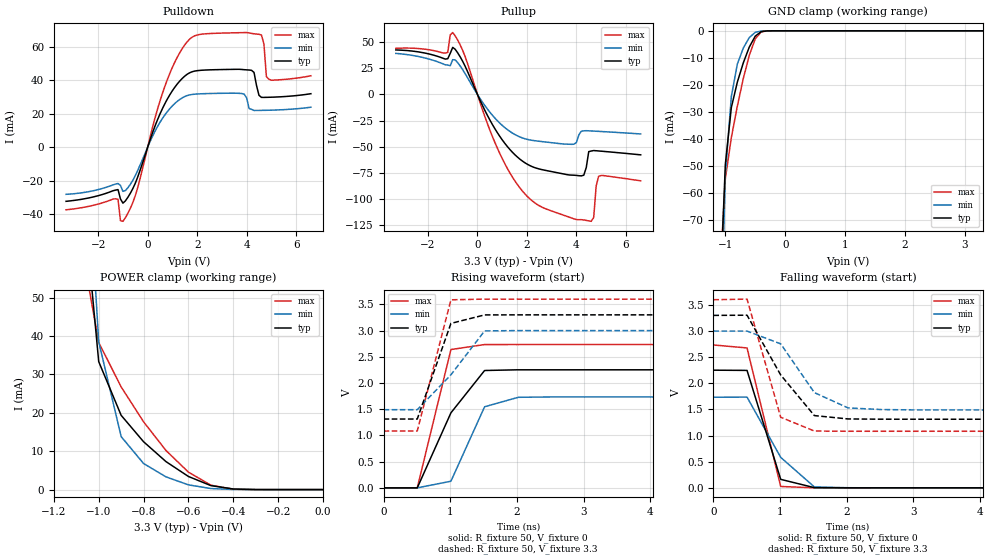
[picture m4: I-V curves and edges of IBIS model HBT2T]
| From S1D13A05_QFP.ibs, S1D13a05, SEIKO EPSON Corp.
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[Model]   HBT2T
Model_type I/O
Enable Active-Low
Polarity Non-Inverting
Vinh=2.0
Vinl=0.8
Vref=0
Vmeas=1.65
Rref=500
Cref=100pf
C_comp   5p   4p   6p
[Temperature Range] 25   85   -40
[Voltage Range]   3.3   3.0   3.6
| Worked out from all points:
|   slope of the pulldown table from 0 to 0.495 V, typ, clamps not added: 25.1 ohm
|   slope of the pullup table from 0 to 0.495 V, typ, clamps not added: 20.5 ohm
|   GND clamp passes 1 mA (typ) near -0.44 V on its own axis
|   POWER clamp passes 1 mA (typ) near -0.50 V on its own axis
|   falling waveform, R_fixture 50, V_fixture 0: 20-80 % time 327ps typ, 563ps min, 313ps max; typ from 2.25 V to 0 V
|   falling waveform, R_fixture 50, V_fixture 3.3: 20-80 % time 620ps typ, 525ps min, 337ps max; typ from 3.3 V to 1.31 V
|   rising waveform, R_fixture 50, V_fixture 0: 20-80 % time 578ps typ, 370ps min, 314ps max; typ from 0 V to 2.25 V
|   rising waveform, R_fixture 50, V_fixture 3.3: 20-80 % time 330ps typ, 603ps min, 305ps max; typ from 1.31 V to 3.3 V
[Pullup]
-3.3V     42.64mA    39.34mA    44.21mA
-1.3V     33.9mA     28.39mA    39.63mA
-1V       45.11mA    33.33mA    59.3mA
1V        -43.46mA   -29.62mA   -61.38mA
2.5V      -71.44mA   -44.88mA   -106.7mA
3.9V      -77.38mA   -47.7mA    -119.2mA
4.3V      -77.38mA   -34.88mA   -120.3mA
4.6V      -54.24mA   -34.99mA   -121.6mA
4.7V      -53.77mA   -35.12mA   -117.9mA
4.8V      -53.97mA   -35.26mA   -87.72mA
4.9V      -54.17mA   -35.39mA   -78.51mA
6.6V      -57.89mA   -37.87mA   -82.79mA
[Pulldown]
-3.3V     -32.36mA   -28.18mA   -37.42mA
-1.2V     -25.35mA   -21.72mA   -31.11mA
-1V       -33.45mA   -26.41mA   -44.3mA
-500mV    -21.54mA   -17mA      -28.96mA
800mV     28.85mA    21.31mA    40.54mA
1.8V      45.04mA    31.48mA    65.72mA
3.8V      46.4mA     32.04mA    68.39mA
4.2V      45.88mA    22.57mA    67.94mA
4.6V      29.73mA    21.96mA    67mA
4.8V      29.74mA    22.01mA    42.16mA
4.9V      29.78mA    22.05mA    40.55mA
6.6V      31.92mA    23.85mA    42.62mA
[GND Clamp]
-3.3V     -4.024A    -3.586A    -4.684A
-1.1V     -104.6mA   -131.9mA   -94.35mA
-1V       -49.45mA   -53.21mA   -54.75mA
-900mV    -28.43mA   -24.36mA   -39.57mA
-800mV    -19.03mA   -12.35mA   -27.94mA
-700mV    -11.86mA   -6.392mA   -17.67mA
-600mV    -6.019mA   -2.491mA   -9.09mA
-500mV    -1.963mA   -559.1uA   -2.967mA
-400mV    -291.4uA   -72.87uA   -373.1uA
-300mV    -21.59uA   -6.634uA   -18.01uA
3.3V      1.101nA    2.93uA     42.72pA
[POWER Clamp]
-3.3V     4.048A     3.62A      4.667A
-1.1V     95.68mA    136.1mA    70.93mA
-1V       33.32mA    38.49mA    38.31mA
-900mV    19.33mA    13.79mA    26.73mA
-800mV    12.45mA    6.785mA    17.64mA
-700mV    7.275mA    3.309mA    10.16mA
-600mV    3.411mA    1.231mA    4.531mA
-500mV    1.036mA    277uA      1.153mA
-400mV    155.5uA    36.16uA    108uA
0V        1.101nA    2.479nA    111.9pA
[Falling Waveform]
R_fixture=50
V_fixture=0
V_fixture_min=0
V_fixture_max=0
0s        2.252V     1.734V     2.734V
505.1ps   2.247V     1.736V     2.677V
1.01ns    162.3mV    583mV      26.1mV
1.515ns   3.399mV    17.27mV    244.8uV
2.02ns    -474.6uV   1.886mV    -11.26uV
50ns      -962.1nV   2.018uV    0V
[Falling Waveform]
R_fixture=50
V_fixture=3.3
V_fixture_min=3.0
V_fixture_max=3.6
0s        3.3V       3V         3.6V
505.1ps   3.304V     3V         3.611V
1.01ns    2.16V      2.755V     1.351V
1.515ns   1.383V     1.823V     1.087V
2.02ns    1.318V     1.529V     1.082V
2.525ns   1.313V     1.498V     1.083V
3.03ns    1.313V     1.491V     1.082V
50ns      1.313V     1.491V     1.082V
[Rising Waveform]
R_fixture=50
V_fixture=0
V_fixture_min=0
V_fixture_max=0
0s        0V         0V         0V
505.1ps   -18.73uV   -10.16uV   334.6uV
1.01ns    1.431V     126.8mV    2.639V
1.515ns   2.239V     1.547V     2.734V
2.02ns    2.252V     1.727V     2.734V
2.525ns   2.252V     1.734V     2.734V
50ns      2.252V     1.734V     2.734V
[Rising Waveform]
R_fixture=50
V_fixture=3.3
V_fixture_min=3.0
V_fixture_max=3.6
0s        1.313V     1.491V     1.082V
505.1ps   1.313V     1.491V     1.086V
1.01ns    3.137V     2.157V     3.587V
1.515ns   3.299V     2.994V     3.6V
50ns      3.3V       3V         3.6V
[Ramp]
R_load=50
dV/dt_r   1.351E+0/2.417E-10   1.041E+0/3.407E-10   1.640E+0/1.786E-10
dV/dt_f   1.192E+0/3.609E-10   9.054E-1/5.150E-10   1.511E+0/2.682E-10
